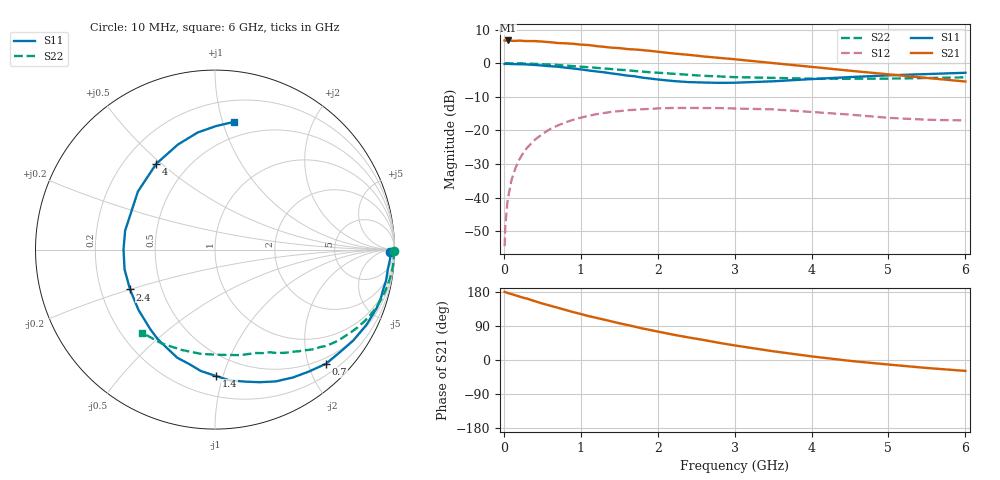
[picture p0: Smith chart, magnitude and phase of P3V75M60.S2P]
! SIEMENS Small Signal Semiconductors
! BFP181
! Si NPN RF Bipolar Junction Transistor in SOT143
! VCE = 0.75 V  IC = 0.6 mA
! Common Emitter S-Parameters:  March  1996
# GHz  S  MA  R  50
!  f  S11  S21  S12  S22
! GHz  MAG  ANG  MAG  ANG  MAG  ANG  MAG  ANG
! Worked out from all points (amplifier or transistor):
!   36 points, 10 MHz to 6 GHz, reference 50 ohm
!   highest |S21| = 6.8 dB at 50 MHz (marker M1)
!   |S21| within 3 dB of that: start of sweep to 1.862 GHz
!   unconditionally stable (mu >= 1): 3.394 GHz to end of sweep
!   at 250 MHz: K = 0.09, MSG = 16.7 dB, |S12| = -26.8 dB
!   at 1.4 GHz: K = 0.48, MSG = 9.6 dB, |S12| = -14.5 dB
!   at 6 GHz: K = 1.59, MAG = 1.3 dB, |S12| = -17.0 dB
!   S11 on the Smith chart (normalised r, x): 10 MHz: 63, -29; 700 MHz: 0.39, -2.31; 1.4 GHz: 0.34, -0.95; 2.4 GHz: 0.33, -0.20; 4 GHz: 0.33, +0.48; 6 GHz: 0.37, +1.09
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0.01  0.9741 -0.7  2.176 179.8  0.0019 86.9  0.9995 -0.3
0.02  0.9757 -1.4  2.153 179.4  0.0039 85.8  0.9981 -0.7
0.05  0.9774 -2.9  2.177 176.9  0.0094 90.8  0.9968 -1.8
0.1  0.9691 -6.7  2.153 173.9  0.0183 84.3  0.9971 -3.4
0.15  0.969 -10.2  2.144 170.8  0.0274 82.3  0.995 -5.1
0.25  0.963 -16.6  2.141 164.5  0.0457 78.5  0.9898 -8.5
0.4  0.9422 -26.4  2.13 155.3  0.0723 71.6  0.9775 -13.4
0.5  0.922 -33.3  2.096 149.1  0.0882 66.5  0.9666 -16.7
0.7  0.887 -45.8  1.993 137.9  0.1185 58.0  0.9385 -22.9
0.9  0.8345 -58.6  1.942 126.5  0.144 49.5  0.9051 -28.6
1.1  0.7791 -71.5  1.861 116.0  0.1647 41.8  0.869 -33.8
1.4  0.7046 -89.5  1.7 101.9  0.1885 31.2  0.8172 -41.1
1.5  0.6812 -96.6  1.677 97.0  0.1935 28.3  0.7979 -42.9
1.8  0.6098 -116.1  1.566 83.3  0.2063 20.1  0.7492 -48.5
2.2  0.5429 -141.7  1.396 66.9  0.2158 9.8  0.6963 -55.6
2.4  0.523 -154.9  1.332 59.6  0.2165 5.1  0.6719 -59.1
3  0.5118 168.1  1.144 38.5  0.2119 -6.4  0.6197 -68.4
3.5  0.5378 143.0  1.003 23.1  0.2055 -13.4  0.6047 -76.5
4  0.5794 124.4  0.881 9.6  0.1883 -19.3  0.5875 -86.5
4.5  0.621 109.4  0.772 -2.3  0.1717 -23.6  0.5863 -97.3
5.5  0.6888 89.4  0.603 -21.1  0.1442 -22.2  0.6018 -119.8
6  0.7199 81.4  0.534 -28.8  0.1406 -19.0  0.6154 -131.2
